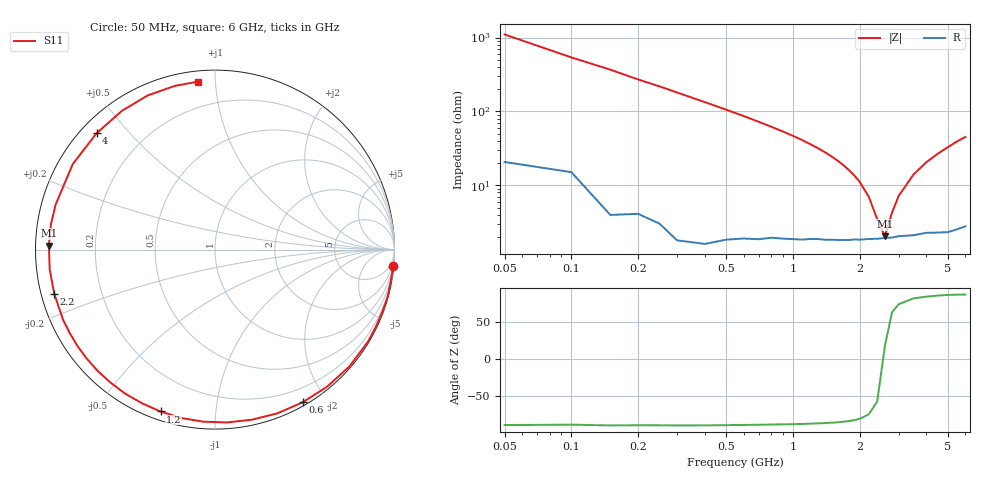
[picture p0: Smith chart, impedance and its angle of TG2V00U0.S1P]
! SIEMENS Discrete & RF Semiconductors
! BAT64
! Si Schottky Diode in SOT23
! VR = 2 V
! S-Parameters:  February  1997
# GHz  S  MA  R  50
!  f  S11
! GHz  MAG  ANG
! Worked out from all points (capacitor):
!   34 points, 50 MHz to 6 GHz, reference 50 ohm
!   read as one part to ground: C = 2.89 pF near 50 MHz
!   lowest |Z| = 2.03 ohm at 2.6 GHz (marker M1)
!   series resonance near 2.565 GHz, so ESL is about 1.3 nH
!   S11 on the Smith chart (normalised r, x): 50 MHz: 0, -22; 600 MHz: 0.04, -1.73; 1.2 GHz: 0.04, -0.72; 2.2 GHz: 0.04, -0.13; 4 GHz: 0.05, +0.41; 6 GHz: 0.06, +0.90
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0.05  0.9983 -5.2
0.15  0.9971 -15.5
0.3  0.9949 -31.0
0.4  0.9921 -41.0
0.5  0.9866 -50.7
0.6  0.9811 -60.1
0.7  0.9763 -69.2
0.8  0.9697 -77.9
0.9  0.9653 -86.1
1  0.9609 -93.9
1.1  0.9569 -101.4
1.2  0.9517 -108.6
1.4  0.9456 -121.9
1.6  0.9404 -134.0
1.7  0.9378 -139.7
1.9  0.9333 -150.3
2  0.9325 -155.2
2.2  0.929 -164.7
2.4  0.9275 -173.3
2.6  0.9255 178.6
2.8  0.9249 171.3
3  0.9228 164.3
3.5  0.9248 149.0
4  0.9251 135.5
4.5  0.9312 123.8
5  0.9372 113.5
5.5  0.9391 103.8
6  0.9405 95.9
